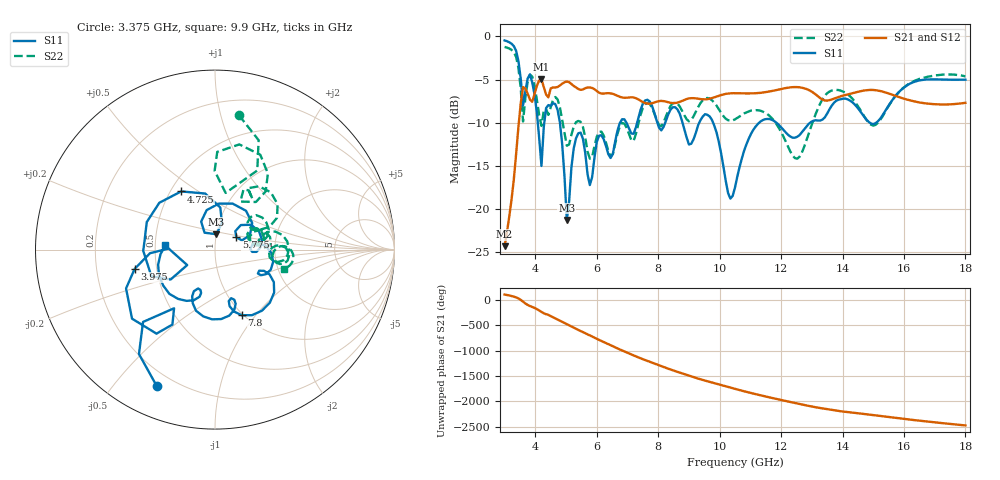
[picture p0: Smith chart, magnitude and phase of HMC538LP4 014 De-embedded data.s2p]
! Chelmsford, MA 01824
! http://www.hittite.com
! Tel: 978-250-3343
! Fax: 978-250-3373
! Device  :  HMC538LP4
! Description:  600 Analog Phase Shifter
! Frequency  :  6.0 GHz - 15.0 GHz
! Package  :  LP4  - 4x4 mm Quad Flatpack No-Lead (QFN) Plastic Package: 24 pin
! Ports  :  2 RF, 1 DC
!  Pin  3  = Rfin  = Port 1
!  Pin  16  = Rfout = Port 2
!  pin  21  = vCTL
! Voltages:  VCTL  = 0 to 5.0 Volts
! Currents :  Vb(V)  Vd(V)  Ib(mA)  Id(mA)
!  0.00  1.40  0.000000	0.491626
! Data:  The device was measured on evaluation board 111296-1.
!  Data was collected using a calibrated network analyzer.
!  The evaluation circuit board was modeled and simulated.This was use
!  to removed the evaluation board circuit from the measured data.
!  The reference plane is the center of the package pin.
! Misc:  Lot #
!Date Measured:  03 - 11 -2009
! Date:  03 - 17 -2009
! Note:
!  Hittite Microwave supplies this data as a sample of measured data at the
!  package pin for this package product.  Your particular data for this product
!  may vary.
!  Data was taken at 25 degrees C.
!  Hittite Microwave reserves the right to change this data at anytime.
# MHz S MA R 50
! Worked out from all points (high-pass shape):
!   201 points, 3 GHz to 18 GHz, reference 50 ohm
!   highest |S21| = -4.97 dB at 4.2 GHz (marker M1); lowest = -24.3 dB at 3 GHz (marker M2)
!   |S21| within 3 dB of the highest: 3.519 GHz to end of sweep
!   lowest |S11| = -21.3 dB at 5.025 GHz (marker M3), VSWR 1.19, Z = 50.1 + j8.66 ohm
!   |S11| at or under -10 dB: 4.801 GHz to 6.759 GHz (1.958 GHz wide, 33.9 % of centre); 9.786 GHz to 11.29 GHz (1.503 GHz wide, 14.3 % of centre); 11.85 GHz to 12.95 GHz (1.101 GHz wide, 8.88 % of centre)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
!   |S22| runs from -14.2 to -1.2 dB; largest |S21 - S12| = 0.0013
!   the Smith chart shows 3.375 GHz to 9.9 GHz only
!   S11 on the Smith chart (normalised r, x): 3.375 GHz: 0.14, -0.65; 3.975 GHz: 0.37, -0.10; 4.725 GHz: 0.57, +0.43; 5.775 GHz: 1.26, +0.17; 7.8 GHz: 0.98, -0.85; 9.9 GHz: 0.57, +0.03
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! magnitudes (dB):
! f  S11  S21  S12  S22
! 3 GHz  -0.5  -24.3  -24.3  -1.2
! 3.375 GHz  -1.7  -13.6  -13.6  -2.4
! 3.6 GHz  -8.0  -5.9  -5.9  -9.9
! 3.975 GHz  -6.7  -6.6  -6.6  -5.7
! 4.2 GHz  -15.0  -5.0  -5.0  -10.4
! 4.35 GHz  -8.3  -6.7  -6.7  -8.4
! 4.725 GHz  -8.5  -5.9  -5.9  -7.3
! 5.025 GHz  -21.3  -5.2  -5.2  -12.7
! 5.25 GHz  -13.0  -5.7  -5.7  -10.5
! 5.55 GHz  -11.9  -6.1  -6.1  -10.5
! 5.775 GHz  -17.2  -5.9  -5.9  -14.2
! 6.075 GHz  -11.5  -6.5  -6.5  -11.1
! 6.45 GHz  -14.1  -6.6  -6.6  -13.9
! 7.8 GHz  -8.1  -7.7  -7.8  -8.3
! 8.025 GHz  -10.6  -7.5  -7.5  -10.3
! 9.9 GHz  -11.2  -7.0  -7.0  -8.0
! 10.5 GHz  -17.5  -6.6  -6.6  -9.6
! 11.32 GHz  -9.9  -6.5  -6.5  -8.6
! 12.53 GHz  -11.6  -5.9  -5.9  -14.2
! 13.05 GHz  -9.8  -6.5  -6.5  -9.7
! 15.53 GHz  -7.9  -6.6  -6.6  -7.9
! 18 GHz  -5.0  -7.7  -7.7  -4.6
